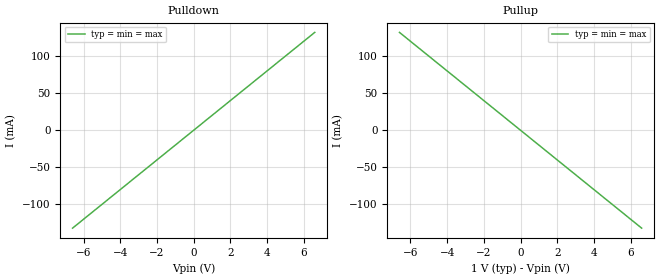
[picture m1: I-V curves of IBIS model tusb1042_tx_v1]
[IBIS Ver]   5.1
[File Name]   tusb1042_rxtx2.ibs
[File Rev]   1.0
[Component]   tusb1046_rxtx1
[Manufacturer] My Company
[Package]
R_pkg  0.0   NA   NA
L_pkg  0.0   NA   NA
C_pkg  0.0   NA   NA
[Pin]   signal_name   model_name   R_pin L_pin  C_pin
1p   tusb1042_tx_v1_p   tusb1042_tx_v1
1n   tusb1042_tx_v1_n   tusb1042_tx_v1
2p   tusb1042_rx2_2p   tusb1042_rx2
2n   tusb1042_rx2_2n   tusb1042_rx2
[Diff_Pin] inv_pin vdiff tdelay_typ tdelay_min tdelay_max
1p   1n   NA   NA   NA   NA
2p   2n   NA   NA   NA   NA
[Model] tusb1042_rx2
Model_type Input
C_comp 0p 0p 0p
Vinh = 0.25
Vinl = -0.25
[Temperature_Range] 25 125 0
[Voltage Range] 1.0 1.0 1.0
[Algorithmic Model]
Executable Windows_cl17.00.50727.1_64 tusb1042_rx2_x64.dll tusb1042_rx2.ami
[End Algorithmic Model]
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| Models and submodels in the file (2): tusb1042_tx_v1 (Output), tusb1042_rx2 (Input)
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[Model] tusb1042_tx_v1
Model_type Output
C_comp 0p 0p 0p
Cref = 0
Vref = 0.5
Rref = 50
Vmeas = 0.5
[Temperature_Range] 25 125 0
[Voltage Range] 1.0 1.0 1.0
[Algorithmic Model]
Executable Windows_cl17.00.50727.1_64 tusb1042_tx_v1_x64.dll tusb1042_tx_v1.ami
[End Algorithmic Model]
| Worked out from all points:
|   slope of the pulldown table from 0 to 0.15 V, typ, clamps not added: 50 ohm
|   slope of the pullup table from 0 to 0.15 V, typ, clamps not added: 50 ohm
[Pulldown]
-6.6V     -132mA     -132mA     -132mA
0V        0A         0A         0A
6.6V      132mA      132mA      132mA
[Pullup]
-6.6V     132mA      132mA      132mA
0V        0A         0A         0A
6.6V      -132mA     -132mA     -132mA
[GND Clamp]
-6.6V     0A         0A         0A
0V        0A         0A         0A
6.6V      0A         0A         0A
[Power Clamp]
-6.6V     0A         0A         0A
0V        0A         0A         0A
6.6V      0A         0A         0A
[Ramp]
dV/dt_r 0.3/1.5p 0.3/1.5p 0.3/1.5p
dV/dt_f 0.3/1.5p 0.3/1.5p 0.3/1.5p
